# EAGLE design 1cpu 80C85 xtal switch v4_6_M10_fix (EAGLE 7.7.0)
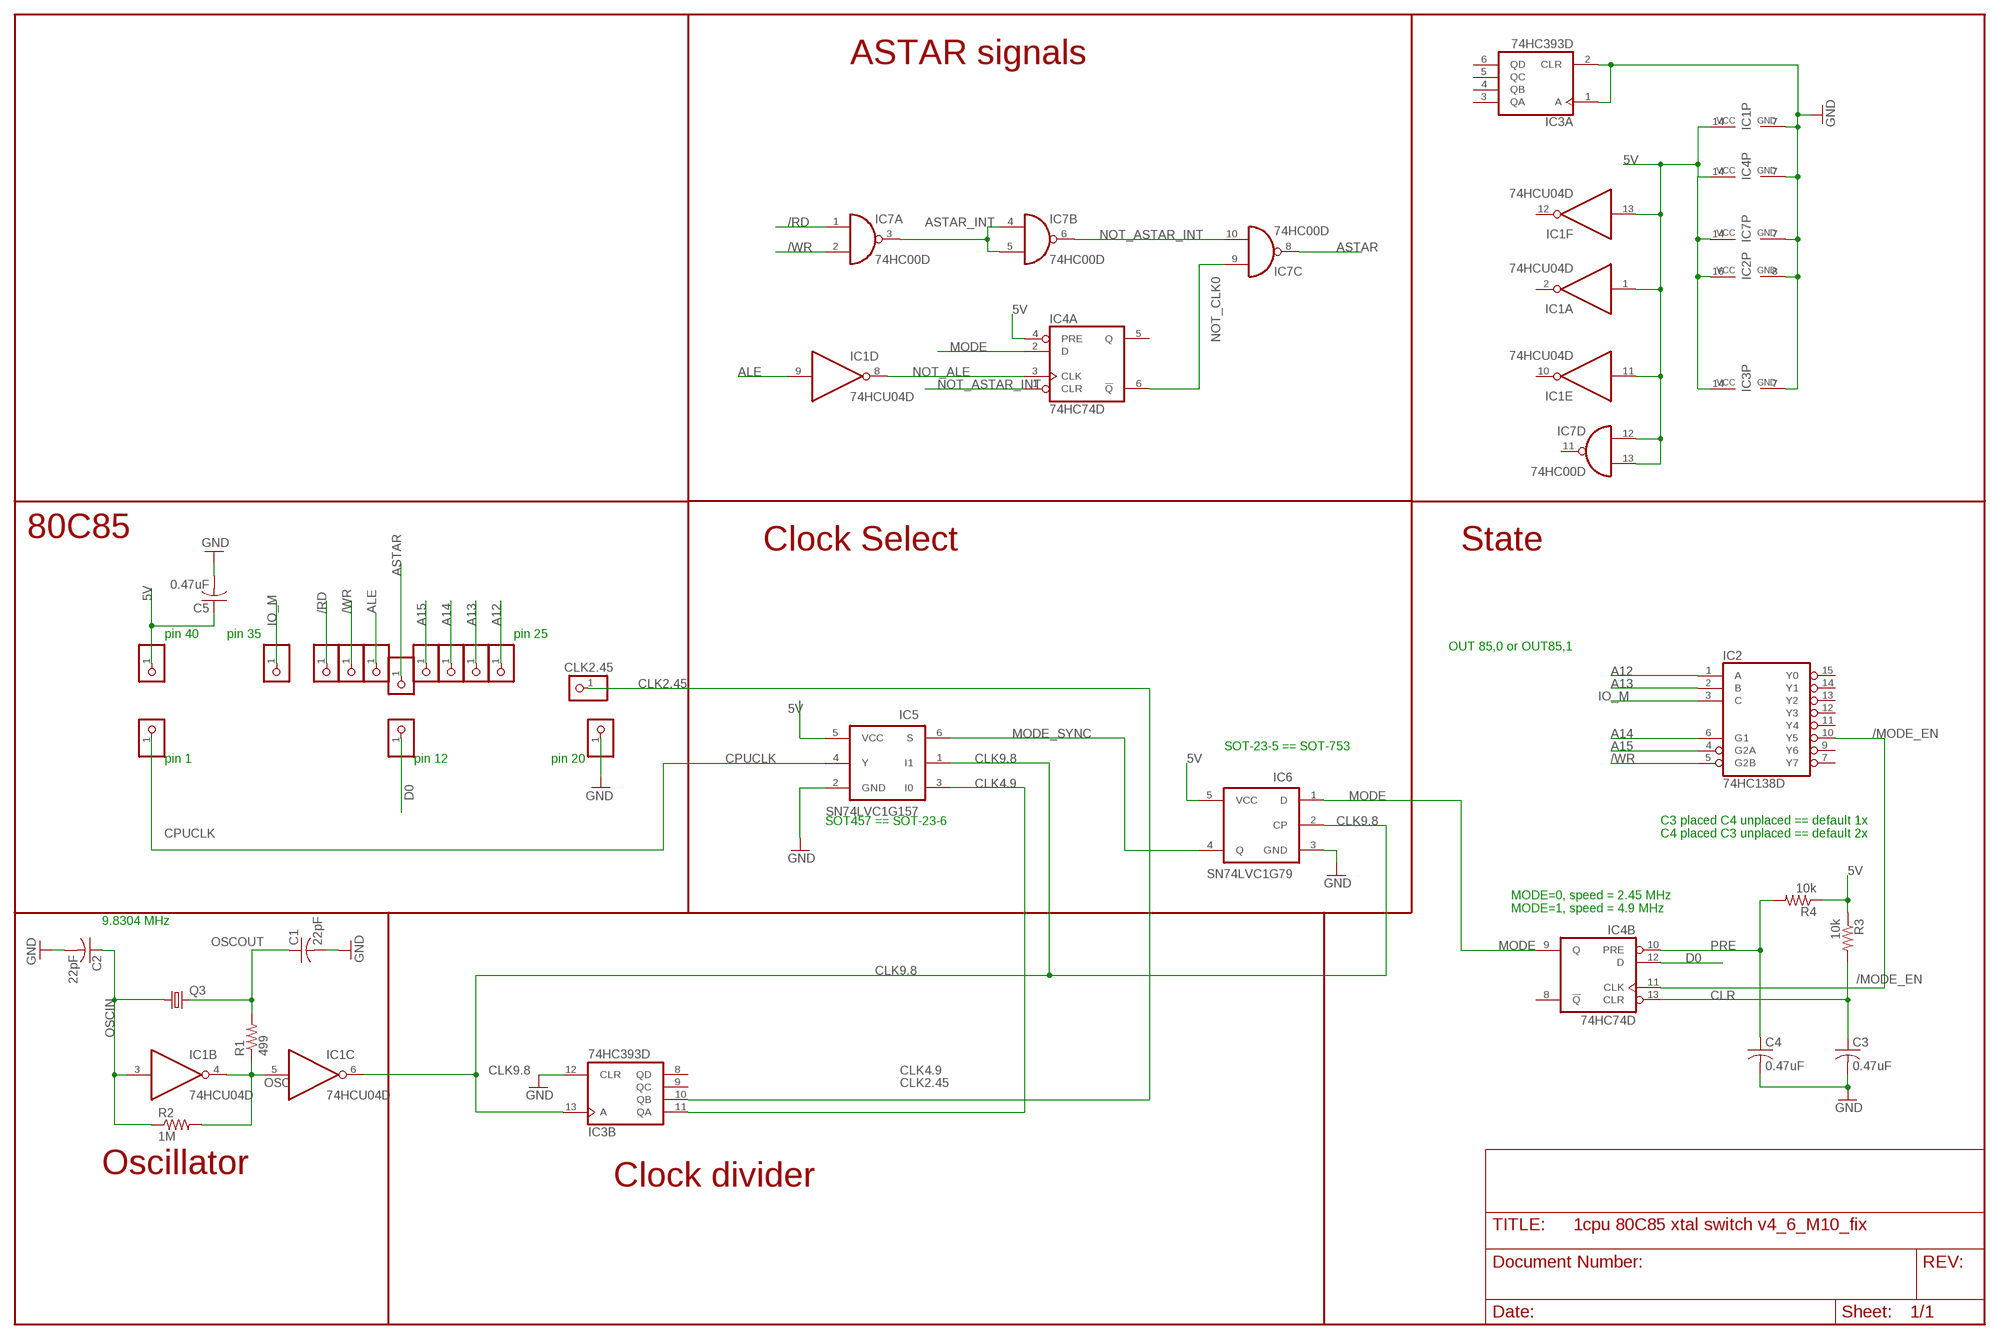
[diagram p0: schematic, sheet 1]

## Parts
5V  PINHD-1X1  [1X01]
5V1  PINHD-1X1  [1X01]
5V2  PINHD-1X1  [1X01]
5V3  PINHD-1X1  [1X01]
5V5  PINHD-1X1  [1X01]
5V7  PINHD-1X1  [1X01]
5V8  PINHD-1X1  [1X01]
5V9  PINHD-1X1  [1X01]
5V10  PINHD-1X1  [1X01]
C1  22pF  C-US025-025X050  [C025-025X050]
C2  22pF  C-US025-025X050  [C025-025X050]
C3  0.47uF  C-US025-025X050  [C025-025X050]
C4  0.47uF  C-US025-025X050  [C025-025X050]
C5  0.47uF  C-US025-025X050  [C025-025X050]
GND5  PINHD-1X1  [1X01]
GND8  PINHD-1X1  [1X01]
GND10  PINHD-1X1  [1X01]
IC1  74HCU04D  74HC04D  [SO14]
IC2  74HC138D  [SO16]
IC3  74HC393D  [SO14]
IC4  74HC74D  [SO14]
IC5  SN74LVC1G157  [SOT23-6]
IC6  SN74LVC1G79  [SOT23-5]
IC7  74HC00D  [SO14]
Q3  CRYSTALHC49S  [HC49/S]
R1  499  R-US_0204/5  [0204/5]
R2  1M  R-US_0204/5  [0204/5]
R3  10k  R-US_0204/5  [0204/5]
R4  10k  R-US_0204/5  [0204/5]
SEL2  PINHD-1X1  [1X01]
SEL3  PINHD-1X1  [1X01]

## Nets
5V: 5V.1 C5.1 IC1.1(A:I) IC1.11(E:I) IC1.13(F:I) IC1.14(P:VCC) IC2.16(VCC) IC3.14(P:VCC) IC4.4(A:PRE) IC4.14(P:VCC) IC5.5(VCC) IC6.5(VCC) IC7.12(D:I0) IC7.13(D:I1) IC7.14(P:VCC) R3.1 R4.1
/MODE_EN: IC2.10(Y5) IC4.11(B:CLK)
/RD: 5V5.1 IC7.1(A:I0)
/WR: 5V3.1 IC2.5(G2B) IC7.2(A:I1)
A12: 5V10.1 IC2.1(A)
A13: 5V9.1 IC2.2(B)
A14: 5V8.1 IC2.6(G1)
A15: 5V7.1 IC2.4(G2A)
ALE: GND10.1 IC1.9(D:I)
ASTAR: IC7.8(C:O) SEL3.1
ASTAR_INT: IC7.3(A:O) IC7.4(B:I0) IC7.5(B:I1)
CLK2.45: IC3.10(B:QB) SEL2.1
CLK4.9: IC3.11(B:QA) IC5.3(I0)
CLK9.8: IC1.6(C:O) IC3.13(B:A) IC5.1(I1) IC6.2(CP)
CLR: C3.1 IC4.13(B:CLR) R3.2
CPUCLK: 5V2.1 IC5.4(Y)
D0: GND8.1 IC4.12(B:D)
GND: C1.2 C2.2 C3.2 C4.2 C5.2 GND5.1 IC1.7(P:GND) IC2.8(GND) IC3.1(A:A) IC3.2(A:CLR) IC3.7(P:GND) IC3.12(B:CLR) IC4.7(P:GND) IC5.2(GND) IC6.3(GND) IC7.7(P:GND)
IO_M: 5V1.1 IC2.3(C)
MODE: IC4.2(A:D) IC4.9(B:Q) IC6.1(D)
MODE_SYNC: IC5.6(S) IC6.4(Q)
NOT_ALE: IC1.8(D:O) IC4.3(A:CLK)
NOT_ASTAR_INT: IC4.1(A:CLR) IC7.6(B:O) IC7.10(C:I1)
NOT_CLK0: IC4.6(A:!Q) IC7.9(C:I0)
OSC: IC1.4(B:O) IC1.5(C:I) R1.1 R2.2
OSCIN: C2.1 IC1.3(B:I) Q3.1 R2.1
OSCOUT: C1.1 Q3.2 R1.2
PRE: C4.1 IC4.10(B:PRE) R4.2
Unconnected: IC1.2(A:O) IC1.10(E:O) IC1.12(F:O) IC2.7(Y7) IC2.9(Y6) IC2.11(Y4) IC2.12(Y3) IC2.13(Y2) IC2.14(Y1) IC2.15(Y0) IC3.3(A:QA) IC3.4(A:QB) IC3.5(A:QC) IC3.6(A:QD) IC3.8(B:QD) IC3.9(B:QC) IC4.5(A:Q) IC4.8(B:!Q) IC7.11(D:O)

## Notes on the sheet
- ASTAR signals
- 80C85
- Clock Select | State
- pin 40 | pin 35 | pin 25
- OUT 85,0 or OUT85,1
- SOT-23-5 == SOT-753
- pin 1 | pin 12 | pin 20
- SOT457 == SOT-23-6
- C3 placed C4 unplaced == default 1x
  C4 placed C3 unplaced == default 2x
- MODE=0, speed = 2.45 MHz
  MODE=1, speed = 4.9 MHz
- 9.8304 MHz
- Oscillator
- Clock divider

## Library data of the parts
5V 5V1-5V3 5V5 5V7-5V10 GND5 GND8 GND10 SEL2 SEL3 = pinhead:PINHD-1X1: PIN HEADER
C1-C5 = resistor:C-US: CAPACITOR, American symbol
IC1 = 74xx-eu:74*04: Hex INVERTER
IC2 = 74xx-eu:74*138: 3-line to 8-line DECODER/DEMULTIPLEXER
IC3 = 74xx-eu:74*393: Dual 4-bit decade and binary COUNTER
IC4 = 74xx-eu:74*74: Dual D type positive edge triggered FLIP FLOP, preset and clear
IC5 = 74LV:SN74LVC1G157: SINGLE 2-INPUT MULTIPLEXER
IC6 = 74LV:SN74LVC1G79: D-TYPE FLIP-FLOP
IC7 = 74xx-eu:74*00: Quad 2-input NAND gate
Q3 = crystal:CRYSTAL: CRYSTAL; OC_FARNELL: 1667008; OC_NEWARK: unknown
R1-R4 = resistor:R-US_: RESISTOR, American symbol

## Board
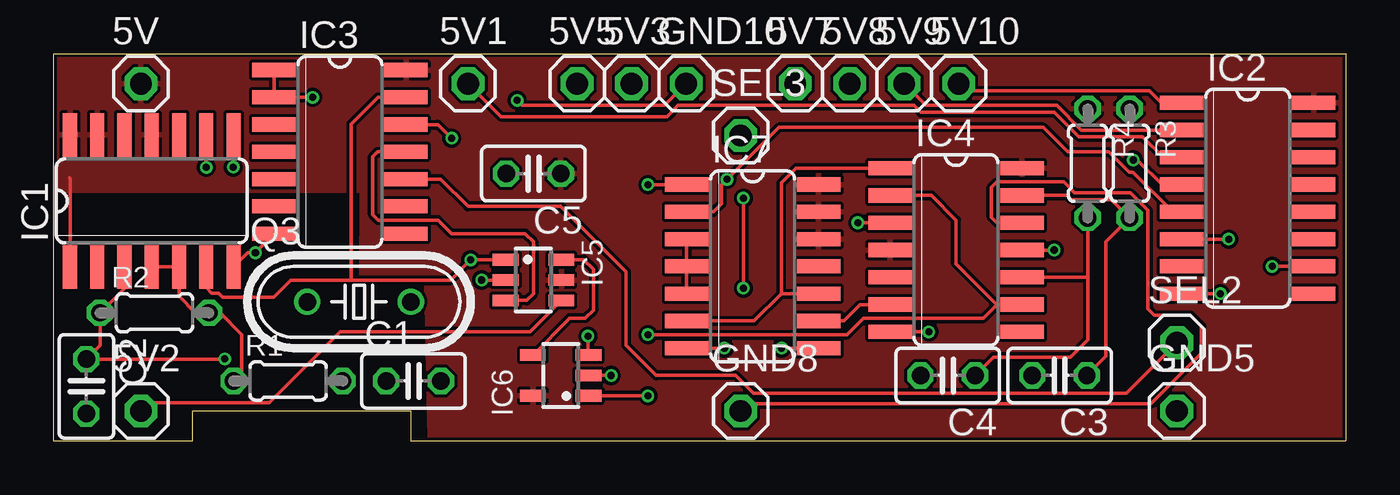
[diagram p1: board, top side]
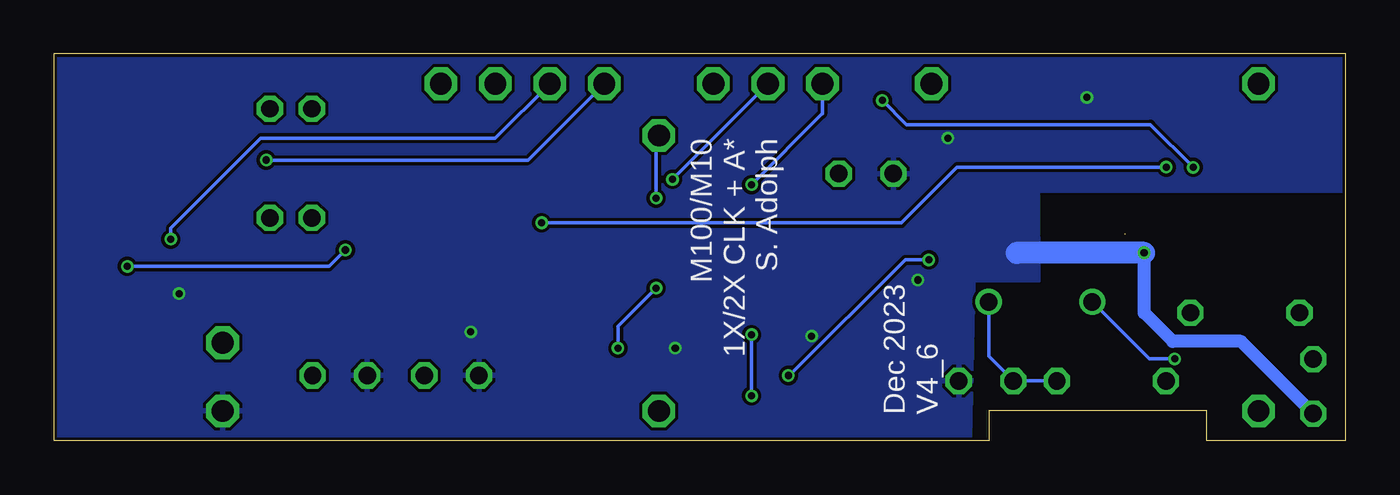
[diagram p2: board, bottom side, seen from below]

Size 60.2 x 18.03 mm. Coordinates in mm from the lower left corner, seen from the top.
Outline: 0,0 6.48,0 6.48,1.4 16.64,1.4 16.64,0 60.2,0 60.2,18.03 0,18.03 0,0
Copper layers (1*16): Top 0.035559375mm / dielectric 1.6mm / Bottom 0.035559375mm
Design rules "oshpark-2layer *": minimum track width 6mil, minimum drill 10mil, track to track 6mil, track to pad 6mil, pad to pad 6mil, via to via 6mil, smd to smd 6mil, copper to edge 6mil, drill to drill 6mil, minimum pad ring 5mil, minimum via ring 5mil, stop-mask expansion 2.5mil, vias tented up to drill 0mil, thermal gap 6mil

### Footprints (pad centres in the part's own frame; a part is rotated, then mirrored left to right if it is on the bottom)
1X01 = drill 1.016 octagon: 1 0,0
C025-025X050 = drill 0.813 octagon: 1 -1.27,0; 2 1.27,0
SO14 = smd 0.66 x 2.032: 1 -3.81,-3.073; 2 -2.54,-3.073; 3 -1.27,-3.073; 4 0,-3.073; 5 1.27,-3.073; 6 2.54,-3.073; 7 3.81,-3.073; 8 3.81,3.073; 9 2.54,3.073; 10 1.27,3.073; 11 0,3.073; 12 -1.27,3.073; 13 -2.54,3.073; 14 -3.81,3.073
SO16 = smd 0.66 x 2.032: 1 -4.445,-3.073; 2 -3.175,-3.073; 3 -1.905,-3.073; 4 -0.635,-3.073; 5 0.635,-3.073; 6 1.905,-3.073; 7 3.175,-3.073; 8 4.445,-3.073; 9 4.445,3.073; 10 3.175,3.073; 11 1.905,3.073; 12 0.635,3.073; 13 -0.635,3.073; 14 -1.905,3.073; 15 -3.175,3.073; 16 -4.445,3.073
SOT23-6 = smd 0.55 x 1.2: 1 -0.95,-1.3; 2 0,-1.3; 3 0.95,-1.3; 4 0.95,1.3; 5 0,1.3; 6 -0.95,1.3
SOT23-5 = smd 0.55 x 1.2: 1 -0.95,-1.3; 2 0,-1.3; 3 0.95,-1.3; 4 0.95,1.3; 5 -0.95,1.3
HC49/S = drill 0.813: 1 -2.413,0; 2 2.413,0
0204/5 = drill 0.813 octagon: 1 -2.54,0; 2 2.54,0

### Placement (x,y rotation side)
5V  4.06,16.64 0 top
5V1  19.3,16.64 0 top
5V2  4.06,1.4 0 top
5V3  26.92,16.64 0 top
5V5  24.38,16.64 0 top
5V7  34.54,16.64 0 top
5V8  37.08,16.64 0 top
5V9  39.62,16.64 0 top
5V10  42.16,16.64 0 top
C1  16.76,2.79 0 top
C2  1.52,2.54 270 top
C3  46.86,3.05 180 top
C4  41.66,3.05 180 top
C5  22.35,12.45 180 top
GND5  52.32,1.4 0 top
GND8  32,1.4 0 top
GND10  29.46,16.64 0 top
IC1  4.57,11.18 0 top
IC2  55.63,11.3 270 top
IC3  13.34,13.46 270 top
IC4  42.04,8.89 270 top
IC5  22.35,7.49 270 top
IC6  23.62,3.05 90 top
IC7  32.56,8.13 270 top
Q3  14.22,6.48 0 top
R1  10.92,2.79 0 top
R2  4.7,5.97 0 top
R3  50.13,12.93 270 top
R4  48.17,12.93 270 top
SEL2  52.32,4.57 0 top
SEL3  32,14.22 0 top

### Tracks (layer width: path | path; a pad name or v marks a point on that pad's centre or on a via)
5V
  Top 0.152: IC1.1 0.76,12.24 0.75,12.26
  pour Top: 0.06,17.95 0.08,11.63 14.31,11.63 14.3,7.44 17.34,7.45 17.49,0.08 60.12,0.09 60.12,17.96
/MODE_EN  (via drill 0.33)
  Top 0.152: IC2.10 v56.77,8.13 | IC4.11 v46.61,8.89
  Bottom 0.152: v56.77,8.13 47.37,8.13 v46.61,8.89
/RD  (via drill 0.33)
  Top 0.152: v27.69,11.94 IC7.1
  Bottom 0.152: 5V5.1 24.38,15.23 24.4,15.23 v27.69,11.94
/WR  (via drill 0.33)
  Top 0.152: 28.68,10.67 IC7.2 30.73,10.67 31.11,11.05 31.11,11.93 v31.37,12.18 33.8,14.61 46.1,14.61 47.24,13.46 49.16,13.46 50.1,12.52 50.28,12.52 52.13,10.67 IC2.5
  Bottom 0.152: 5V3.1 26.92,16.62 v31.37,12.18
A12
  Top 0.152: 5V10.1 42.49,16.31 51.05,16.31 51.61,15.75 IC2.1
A13
  Top 0.152: IC2.2 47.88,14.48 46.74,15.62 40.64,15.62 5V9.1
A14  (via drill 0.33)
  Top 0.152: v54.74,9.4 IC2.6
  Bottom 0.152: 5V8.1 39.62,14.1 50.55,14.1 54.74,9.91 v54.74,9.4
A15  (via drill 0.33)
  Top 0.152: IC2.4 51.64,11.94 50.5,13.08 v50.29,13.08
  Bottom 0.152: 5V7.1 38.1,13.08 v50.29,13.08
ALE  (via drill 0.33)
  Top 0.152: v21.59,15.86 21.83,15.62 28.45,15.62 GND10.1 | IC1.9 v7.11,12.74
  Bottom 0.152: v21.59,15.86 20.46,14.73 9.11,14.73 v7.11,12.74
ASTAR  (via drill 0.33)
  Top 0.152: v32.13,11.3 v32.13,7.11 | 33.9,4.32 v33.91,4.32 IC7.8
  Bottom 0.152: SEL3.1 32.13,14.1 v32.13,11.3 | v32.13,7.11 33.91,5.33 v33.91,4.32
ASTAR_INT
  Top 0.152: IC7.3 IC7.4 IC7.5
CLK2.45
  Top 0.152: SEL2.1 49.96,2.21 32.6,2.21 31.76,3.05 28.07,3.05 26.67,4.45 26.67,7.87 23.62,10.92 19.3,10.92 18.03,12.19 IC3.10
CLK4.9
  Top 0.152: IC5.3 22.04,6.54 22.35,6.86 22.35,9.27 21.97,9.65 18.54,9.65 17.91,10.29 15.11,10.29 14.86,10.54 14.86,13.23 15.09,13.46 IC3.11
CLK9.8  (via drill 0.33)
  Top 0.152: IC1.6 7.1,8.09 7.1,7.15 7.37,6.88 7.68,6.88 7.87,6.69 10.25,6.69 11.05,7.49 13.87,7.49 | 13.87,7.49 18.49,7.49 v19.43,8.43 19.44,8.44 IC5.1 | IC6.2 v25.97,3.05 | 13.87,7.49 13.87,14.76 15.11,16 IC3.13
  Bottom 0.152: v19.43,8.43 20.52,8.43 25.91,3.05 v25.97,3.05
CLR
  Top 0.152: IC4.13 47.23,11.43 47.42,11.24 49.28,11.24 R3.2 49.02,9.28 49.02,3.94 C3.1
CPUCLK
  Top 0.152: 5V2.1 4.45,1.78 10.03,1.78 13.35,5.09 22.2,5.09 IC5.4
D0
  Top 0.152: GND8.1 32.33,1.73 51.12,1.73 53.47,4.08 53.47,5.33 52.96,5.84 51.27,5.84 50.97,6.15 50.97,10.74 50.15,11.56 47.56,11.56 47.05,12.06 43.94,12.06 43.69,11.81 43.69,10.41 43.94,10.16 IC4.12
GND  (via drill 0.33)  (1 unrouted)
  Top 0.152: IC4.7 v40.77,5.08 | IC7.7 v31.24,4.32 | IC2.8 v54.36,6.86 | IC1.7 9.04,8.76 v9.4,8.76 10.26,9.63 | IC3.1 IC3.2 v12.07,16 | IC5.2 v19.94,7.49 | IC6.3 24.89,4.03 v24.89,4.88 | IC3.12 17.91,14.73 v18.54,14.1
  Bottom 0.152: v31.24,4.32 31.41,4.32 31.41,4.33 | v54.36,6.86 54.47,6.86
  Bottom 0.61: C2.2 4.89,4.64 8.06,4.64 9.4,5.97 v9.4,8.76
  Bottom 1.016: v9.4,8.76 15.34,8.76
  pour Bottom: 0.06,17.95 60.12,17.96 60.12,0.09 17.49,0.08 17.34,7.45 14.3,7.44 14.31,11.63 0.08,11.63
IO_M
  Top 0.152: 5V1.1 20.84,15.1 28.56,15.1 29.08,15.62 40.06,15.62 40.07,15.63 40.4,15.3 46.62,15.3 47.75,14.17 50.72,14.17 51.69,13.21 IC2.3
MODE  (via drill 0.33)
  Top 0.152: IC4.9 43.94,6.35 | 43.94,6.35 42.04,8.26 42.04,10.29 40.89,11.43 IC4.2 | v27.69,4.95 36.96,4.95 37.72,5.71 43.31,5.71 43.94,6.35 | v27.69,2.1 v27.68,2.1 IC6.1
  Bottom 0.152: v27.69,4.95 v27.69,2.1
MODE_SYNC
  Top 0.152: IC5.6 24.69,8.44 25.15,7.99 25.15,6.1 24.77,5.71 24.04,5.71 IC6.4 | IC6.4
NOT_ALE  (via drill 0.33)
  Top 0.152: IC4.3 v37.47,10.16 | IC1.8 8.38,13.4 v8.37,12.75
  Bottom 0.152: v8.37,12.75 18.11,12.75 20.7,10.16 v37.47,10.16
NOT_ASTAR_INT
  Top 0.152: IC7.6 32.63,5.59 33.9,6.86 | 33.9,6.86 IC7.10 | IC4.1 34.58,12.7 33.9,12.01 33.9,6.86
NOT_CLK0
  Top 0.152: IC4.6 38.95,6.34 37.57,6.34 36.82,5.59 IC7.9
OSC
  Top 0.152: R1.1 8.76,3.17 8.76,4.95 7.75,5.97 R2.2 6.6,5.97 5.84,6.73 IC1.5 IC1.4
OSCIN  (via drill 0.33)
  Top 0.152: IC1.3 3.3,7.11 R2.1 2.17,4.46 C2.1 7.96,3.81 v7.98,3.82
  Bottom 0.152: v7.98,3.82 9.16,3.82 Q3.1
OSCOUT
  Bottom 0.152: R1.2 C1.1 16.64,3.94 Q3.2
PRE
  Top 0.152: C4.1 43.78,3.9 47.36,3.9 48.17,4.71 48.17,7.59 | R4.2 48.17,7.59 | IC4.10 48.15,7.62 48.17,7.59

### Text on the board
_tsilk: A* | +5 | IO/M | /RD | /WR | ALE | A15 | A14 | A13 | A12 | C5 | 74HCU04 | 74HC393 | R4 | R3 | 74HC138 | 74HC74 | R2 | 1G157 | 74HC00 | C2 | 2.45M | D0 | C4 | C3 | R1 | 1G79 | 2X | 1X | GND | 1 | C1
_bsilk: M100/M10 / 1X/2X CLK + A* / S. Adolph | Dec 2023 / V4_6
